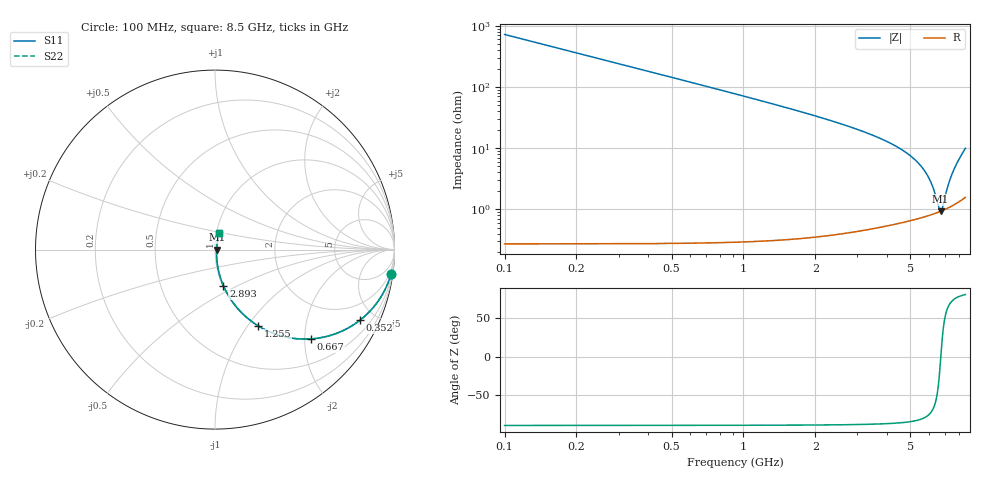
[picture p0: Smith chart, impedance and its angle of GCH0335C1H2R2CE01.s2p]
!Murata Part Number: GCH0335C1H2R2CE01
!These Parameters are Measured in Series Mode Connection
!Data Generated on Mar 13, 2026
!  o--ll--o
!Port1  Port2
!  o------o
!Operation Temp=25[degC], DC Bias Voltage=0[V]
!Freq. Start=100[MHz] Stop=9[GHz] 401[Steps]
# Hz S RI R 50
!Freq.(Hz) S11(Real) S11(Imag) S21(Real) S21(Imag) S12(Real) S12(Imag) S22(Real) S22(Imag)
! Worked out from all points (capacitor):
!   401 points, 100 MHz to 8.5 GHz, reference 50 ohm
!   read as one part in series: C = 2.2 pF near 142 MHz
!   lowest |Z| = 925 mohm at 6.694 GHz (marker M1)
!   series resonance near 6.707 GHz, so ESL is about 260 pH
!   S11 on the Smith chart (normalised r, x): 100 MHz: 1, -14; 352 MHz: 1.01, -4.10; 667 MHz: 1.01, -2.15; 1.255 GHz: 1.01, -1.12; 2.893 GHz: 1.01, -0.43; 8.5 GHz: 1.03, +0.20
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1e8  0.9812 -0.1356  0.0188 0.1356  0.0188 0.1356  0.9812 -0.1356
2.26e8  0.9107 -0.2847  0.0893 0.2847  0.0893 0.2847  0.9107 -0.2847
3.52e8  0.8076 -0.3935  0.1924 0.3935  0.1924 0.3935  0.8076 -0.3935
4.99e8  0.6754 -0.4673  0.3246 0.4673  0.3246 0.4673  0.6754 -0.4673
6.67e8  0.5365 -0.4974  0.4635 0.4974  0.4635 0.4974  0.5365 -0.4974
9.4e8  0.3652 -0.4796  0.6348 0.4796  0.6348 0.4796  0.3652 -0.4796
1.255e9  0.2403 -0.4246  0.7597 0.4246  0.7597 0.4246  0.2403 -0.4246
1.507e9  0.1769 -0.3782  0.8231 0.3782  0.8231 0.3782  0.1769 -0.3782
2.074e9  0.0967 -0.2901  0.9033 0.2901  0.9033 0.2901  0.0967 -0.2901
2.893e9  0.0469 -0.2018  0.9531 0.2018  0.9531 0.2018  0.0469 -0.2018
2.914e9  0.0461 -0.2  0.9539 0.2  0.9539 0.2  0.0461 -0.2
4.3e9  0.0174 -0.1076  0.9826 0.1076  0.9826 0.1076  0.0174 -0.1076
5.119e9  0.0113 -0.068  0.9887 0.068  0.9887 0.068  0.0113 -0.068
5.707e9  0.0092 -0.0424  0.9908 0.0424  0.9908 0.0424  0.0092 -0.0424
6.148e9  0.00867 -0.0238  0.9913 0.0238  0.9913 0.0238  0.00867 -0.0238
6.589e9  0.00895 -0.0051  0.991 0.0051  0.991 0.0051  0.00895 -0.0051
6.694e9  0.00915 -0.000571  0.9909 0.000571  0.9909 0.000571  0.00915 -0.000571
6.799e9  0.00939 0.004  0.9906 -0.004  0.9906 -0.004  0.00939 0.004
7.114e9  0.0105 0.0181  0.9895 -0.0181  0.9895 -0.0181  0.0105 0.0181
7.366e9  0.0118 0.0299  0.9882 -0.0299  0.9882 -0.0299  0.0118 0.0299
7.66e9  0.0138 0.0445  0.9862 -0.0445  0.9862 -0.0445  0.0138 0.0445
8.5e9  0.0245 0.0943  0.9755 -0.0943  0.9755 -0.0943  0.0245 0.0943
